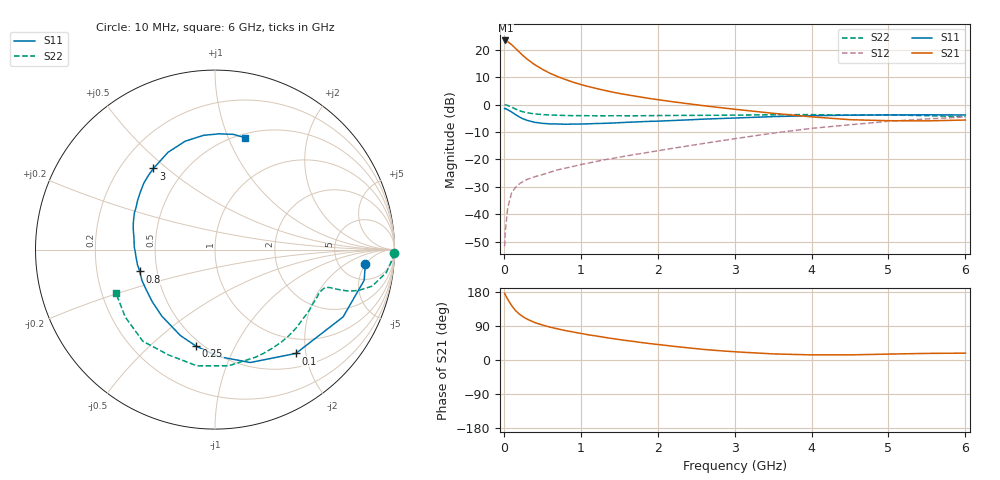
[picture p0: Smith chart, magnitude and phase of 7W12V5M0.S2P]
! Infineon Technologies  Discrete & RF Semiconductors
! BFS17W
! Si NPN RF Bipolar Junction Transistor in SOT323
! VCE = 12 V  IC = 5 mA
! Common Emitter S-Parameters:  August  1999
# GHz  S  MA  R  50
!  f  S11  S21  S12  S22
! GHz  MAG  ANG  MAG  ANG  MAG  ANG  MAG  ANG
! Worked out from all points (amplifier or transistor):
!   36 points, 10 MHz to 6 GHz, reference 50 ohm
!   highest |S21| = 23.4 dB at 20 MHz (marker M1)
!   |S21| within 3 dB of that: start of sweep to 155.5 MHz
!   unconditionally stable (mu >= 1): 595.9 MHz to 2.245 GHz; 5.416 GHz to end of sweep
!   at 250 MHz: K = 0.57, MSG = 23.0 dB, |S12| = -28.1 dB
!   at 1.4 GHz: K = 1.18, MAG = 9.6 dB, |S12| = -19.8 dB
!   at 6 GHz: K = 1.04, MAG = -1.8 dB, |S12| = -4.5 dB
!   S11 on the Smith chart (normalised r, x): 10 MHz: 9, -5; 100 MHz: 0.73, -1.82; 250 MHz: 0.46, -0.71; 800 MHz: 0.40, -0.12; 3 GHz: 0.34, +0.45; 6 GHz: 0.54, +1.15
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0.01  0.8413 -5.6  14.78 176.2  0.0026 86.6  0.9954 -1.1
0.02  0.8486 -11.6  14.78 171.7  0.005 86.8  0.9887 -3.2
0.05  0.8063 -27.7  14.08 160.2  0.0129 77.1  0.9631 -7.6
0.1  0.7333 -52.1  12.42 143.9  0.0241 67.3  0.8991 -13.1
0.15  0.6589 -72.7  10.65 130.8  0.0307 58.8  0.8283 -16.0
0.2  0.5958 -88.3  9.093 121.4  0.0355 55.2  0.776 -17.3
0.25  0.5479 -101.1  7.795 114.0  0.0394 52.1  0.736 -17.8
0.3  0.5163 -111.9  6.797 108.1  0.0429 51.7  0.7096 -18.0
0.4  0.4743 -128.7  5.361 99.0  0.048 51.8  0.6741 -18.3
0.5  0.454 -140.7  4.405 92.4  0.0525 53.1  0.6561 -18.7
0.6  0.4434 -150.0  3.72 86.8  0.0582 55.3  0.6444 -19.5
0.8  0.4366 -163.8  2.864 77.7  0.069 58.4  0.6313 -21.9
0.9  0.4403 -169.1  2.561 73.9  0.0743 60.3  0.6272 -23.3
1.1  0.4449 -178.7  2.131 66.5  0.0854 63.0  0.6252 -26.6
1.4  0.459 170.3  1.702 57.0  0.1029 65.9  0.6247 -32.2
1.6  0.4746 163.8  1.506 51.2  0.1156 67.7  0.6235 -36.3
2.2  0.5114 147.4  1.123 36.3  0.1592 72.1  0.6322 -49.8
3  0.5676 127.2  0.821 21.7  0.238 72.9  0.6405 -69.5
3.5  0.6022 115.7  0.692 16.1  0.3007 70.2  0.6518 -83.3
4.5  0.64 95.7  0.529 13.5  0.4276 59.0  0.6414 -113.7
5.5  0.6502 80.9  0.503 17.4  0.5466 45.5  0.6254 -143.1
6  0.6455 75.1  0.522 18.1  0.5933 38.7  0.6028 -156.4
